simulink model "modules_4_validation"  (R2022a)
settings: Solver=VariableStepAuto  StartTime=0.0  StopTime=10.0  RelTol=1e-3
undefined symbols (not defined in the file or in its folder): magnitude

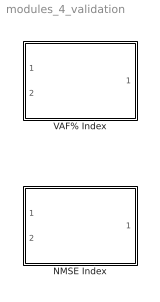
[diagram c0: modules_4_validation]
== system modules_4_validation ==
  NMSE Index : Subsystem
  VAF% Index : Subsystem

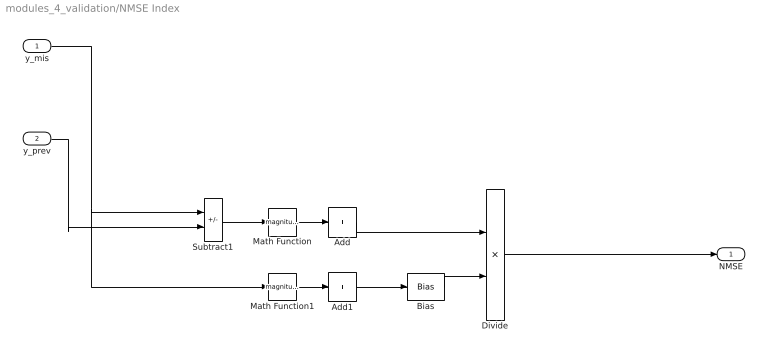
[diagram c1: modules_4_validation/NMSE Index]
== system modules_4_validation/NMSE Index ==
  y_mis : Inport
  y_prev : Inport  Port=2
  Add : Sum  Inputs=+
  Add1 : Sum  Inputs=+
  Bias : Bias  Bias=1e-7
  Divide : Product  Inputs=*/
  Math Function : Math  Operator=magnitude^2
  Math Function1 : Math  Operator=magnitude^2
  Subtract1 : Sum  Inputs=+-
  NMSE : Outport
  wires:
  Math Function/1 -> Add/1
  Bias/1 -> Divide/2
  y_mis/1 -> Math Function1/1, Subtract1/1
  Add1/1 -> Bias/1
  Math Function1/1 -> Add1/1
  Subtract1/1 -> Math Function/1
  Add/1 -> Divide/1
  y_prev/1 -> Subtract1/2
  Divide/1 -> NMSE/1

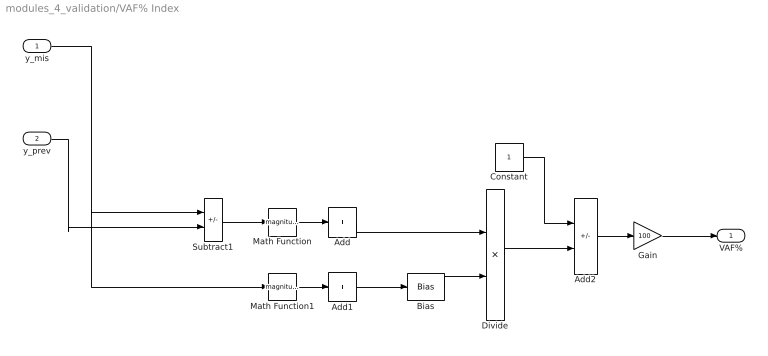
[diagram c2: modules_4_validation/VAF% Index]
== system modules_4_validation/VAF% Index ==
  y_mis : Inport
  y_prev : Inport  Port=2
  Add : Sum  Inputs=+
  Add1 : Sum  Inputs=+
  Add2 : Sum  Inputs=+-
  Bias : Bias  Bias=1e-7
  Constant : Constant
  Divide : Product  Inputs=*/
  Gain : Gain  Gain=100
  Math Function : Math  Operator=magnitude^2
  Math Function1 : Math  Operator=magnitude^2
  Subtract1 : Sum  Inputs=+-
  VAF% : Outport
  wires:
  Add2/1 -> Gain/1
  Math Function/1 -> Add/1
  Bias/1 -> Divide/2
  y_mis/1 -> Math Function1/1, Subtract1/1
  Add1/1 -> Bias/1
  Math Function1/1 -> Add1/1
  Subtract1/1 -> Math Function/1
  Constant/1 -> Add2/1
  Divide/1 -> Add2/2
  Add/1 -> Divide/1
  y_prev/1 -> Subtract1/2
  Gain/1 -> VAF%/1
